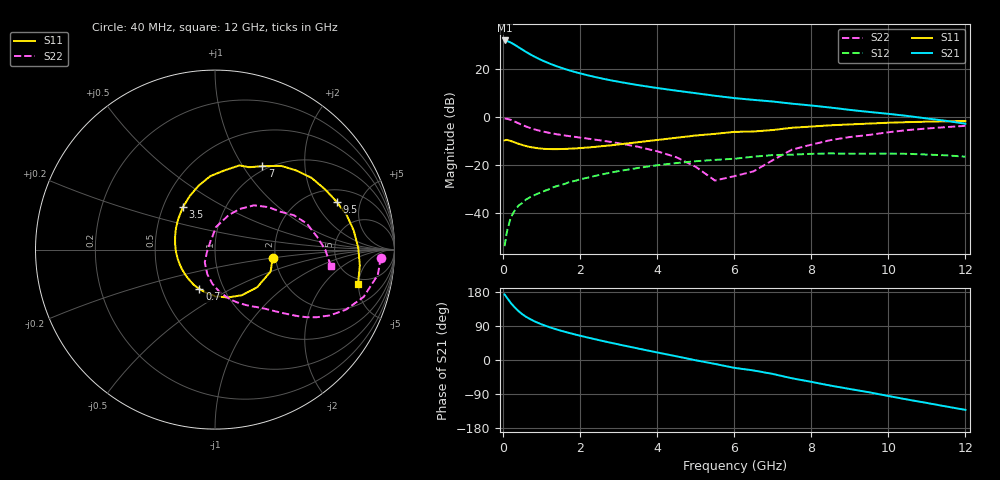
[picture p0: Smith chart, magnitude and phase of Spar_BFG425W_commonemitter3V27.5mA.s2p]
! Filename: 327bfg425.001
! BFG425W Field C1
! V1=8.531E-001V,V2=3.000E+000V, I1=3.718E-004A, I2=2.752E-002A
# GHz  S  MA  R 50
!  S11  S21  S12  S22
!Freq(GHz)  Mag  Ang  Mag  Ang  Mag  Ang  Mag  Ang
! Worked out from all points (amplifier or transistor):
!   44 points, 40 MHz to 12 GHz, reference 50 ohm
!   highest |S21| = 32.0 dB at 40 MHz (marker M1)
!   |S21| within 3 dB of that: start of sweep to 418.9 MHz
!   unconditionally stable (mu >= 1): 1.116 GHz to end of sweep
!   at 700 MHz: K = 0.82, MSG = 29.9 dB, |S12| = -33.6 dB
!   at 2.4 GHz: K = 1.16, MAG = 18.2 dB, |S12| = -24.6 dB
!   at 12 GHz: K = 1.35, MAG = 3.4 dB, |S12| = -16.6 dB
!   S11 on the Smith chart (normalised r, x): 40 MHz: 1.93, -0.20; 700 MHz: 0.77, -0.36; 3.5 GHz: 0.63, +0.33; 7 GHz: 0.94, +1.22; 9.5 GHz: 2.67, +3.04; 12 GHz: 4.23, -4.90
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0.04  0.325 -8.3  39.67 173.0  0.002 62.8  0.925 -2.8
0.1  0.333 -21.5  38.71 164.4  0.004 81.7  0.918 -8.8
0.2  0.315 -41.8  35.92 150.5  0.008 75.8  0.869 -17.7
0.3  0.295 -59.5  32.26 139.0  0.011 71.9  0.803 -24.6
0.4  0.276 -75.4  28.72 129.1  0.014 69.0  0.738 -29.8
0.5  0.26 -89.4  25.52 120.7  0.016 66.7  0.68 -33.7
0.6  0.246 -101.2  22.77 113.8  0.019 65.2  0.631 -36.6
0.7  0.236 -111.5  20.44 108.1  0.021 64.2  0.59 -38.9
0.9  0.222 -129.2  16.82 98.3  0.025 62.8  0.528 -42.4
1.2  0.214 -149.6  13.14 86.8  0.031 60.9  0.466 -46.8
1.6  0.215 -170.8  10.08 74.6  0.04 57.9  0.411 -52.1
2.2  0.23 165.2  7.417 59.2  0.054 52.0  0.353 -60.9
2.8  0.256 145.9  5.829 45.5  0.069 44.8  0.301 -70.7
3.5  0.297 127.0  4.639 30.4  0.086 35.2  0.239 -83.6
4.5  0.368 104.3  3.544 9.8  0.109 20.2  0.144 -107.3
5.5  0.444 83.3  2.773 -10.3  0.127 4.5  0.047 -162.4
6.5  0.497 67.4  2.277 -27.6  0.148 -8.0  0.073 101.7
7  0.534 60.5  2.105 -36.8  0.16 -15.7  0.125 87.8
8.5  0.67 36.7  1.573 -67.6  0.173 -45.0  0.329 48.6
9.5  0.728 21.6  1.274 -85.1  0.171 -61.6  0.422 29.9
10.5  0.78 7.9  1.049 -104.5  0.17 -80.2  0.532 15.8
12  0.819 -13.5  0.724 -131.6  0.148 -109.9  0.653 -8.2
